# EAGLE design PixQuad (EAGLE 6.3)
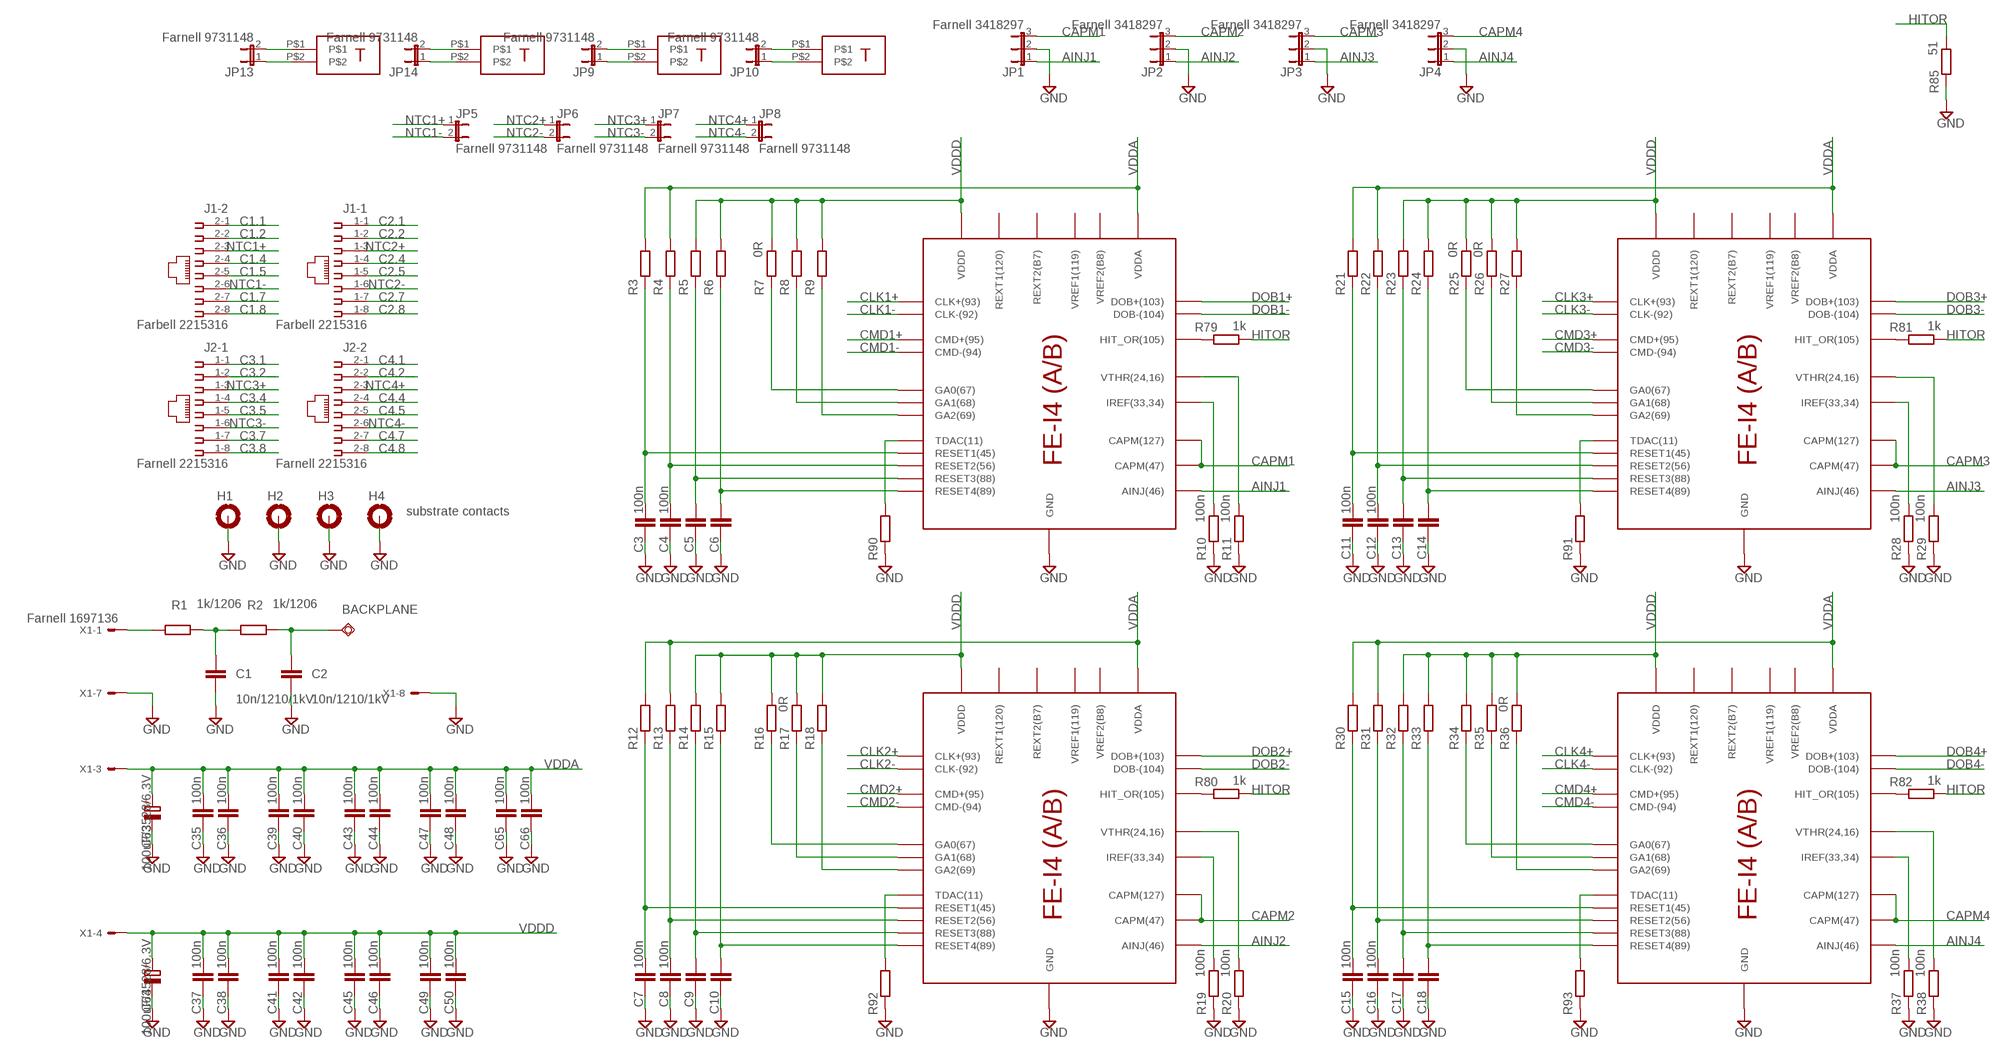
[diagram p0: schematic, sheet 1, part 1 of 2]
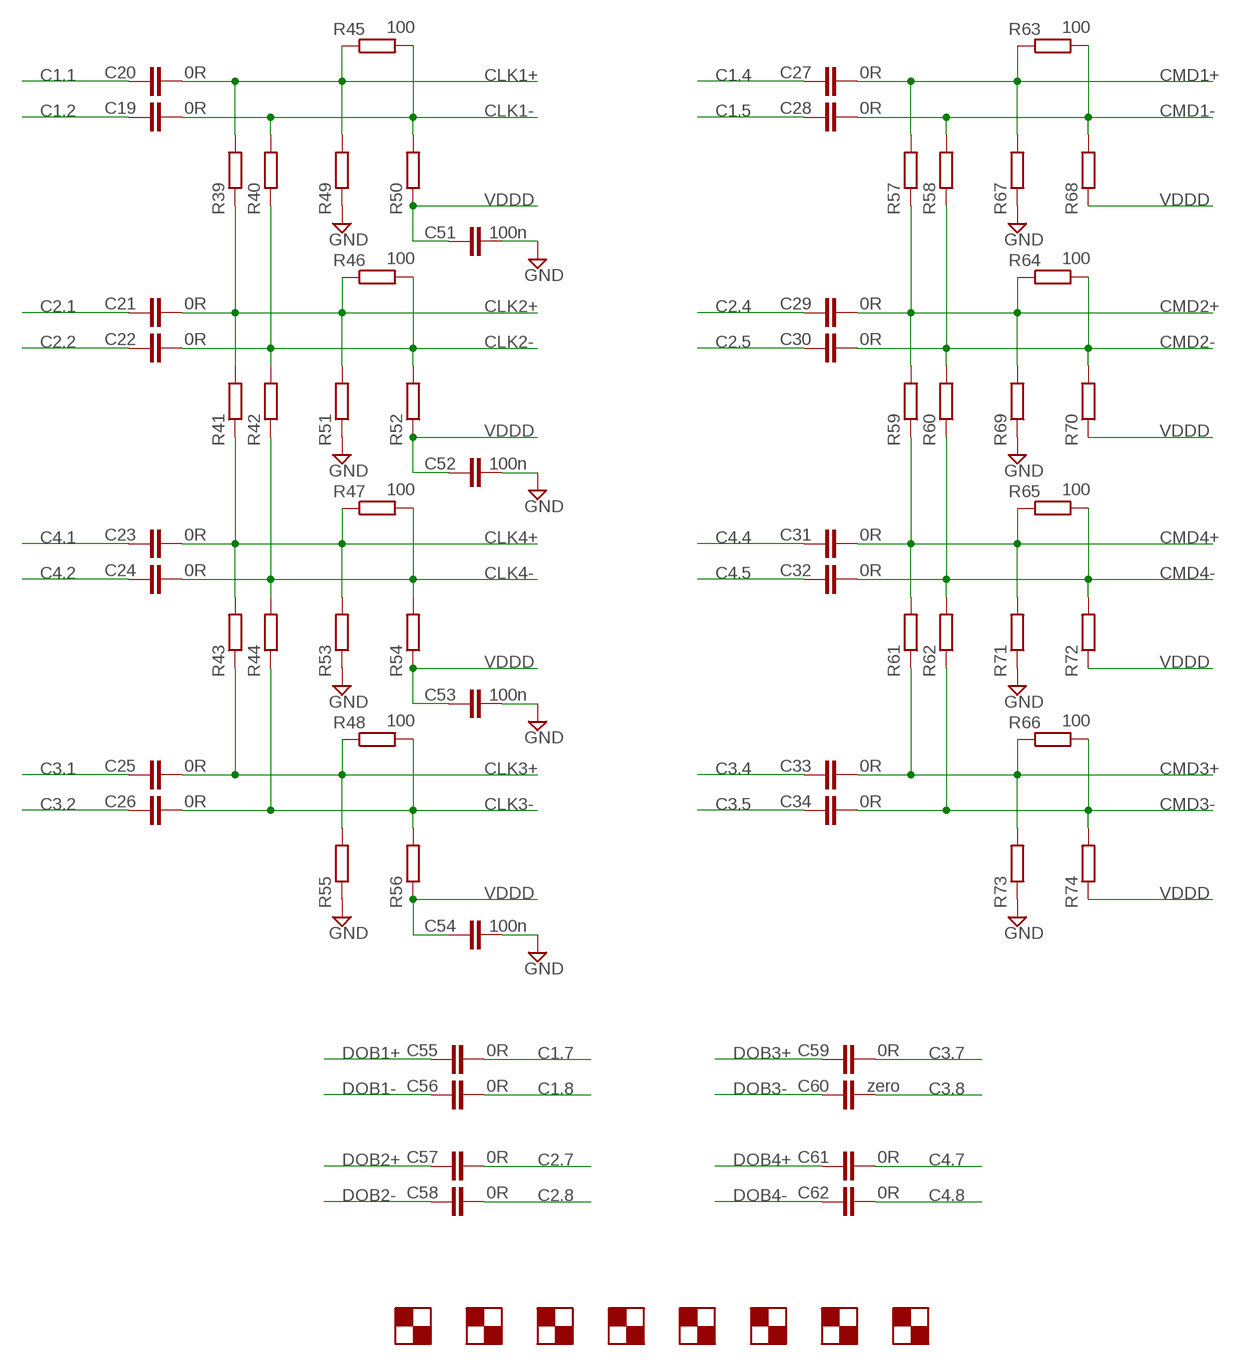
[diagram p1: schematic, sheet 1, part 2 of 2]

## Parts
BACKPLANE  TPSQTP20SQ  [TP20SQ]
C1  10n/1210/1kV  C-EUC1210  [C1210]
C2  10n/1210/1kV  C-EUC1210  [C1210]
C3  100n  C-EUC0402  [C0402]
C4  100n  C-EUC0402  [C0402]
C5  C-EUC0402  [C0402]
C6  C-EUC0402  [C0402]
C7  100n  C-EUC0402  [C0402]
C8  100n  C-EUC0402  [C0402]
C9  C-EUC0402  [C0402]
C10  C-EUC0402  [C0402]
C11  100n  C-EUC0402  [C0402]
C12  100n  C-EUC0402  [C0402]
C13  C-EUC0402  [C0402]
C14  C-EUC0402  [C0402]
C15  100n  C-EUC0402  [C0402]
C16  100n  C-EUC0402  [C0402]
C17  C-EUC0402  [C0402]
C18  C-EUC0402  [C0402]
C19  0R  C-EUC0402  [C0402]
C20  0R  C-EUC0402  [C0402]
C21  0R  C-EUC0402  [C0402]
C22  0R  C-EUC0402  [C0402]
C23  0R  C-EUC0402  [C0402]
C24  0R  C-EUC0402  [C0402]
C25  0R  C-EUC0402  [C0402]
C26  0R  C-EUC0402  [C0402]
C27  0R  C-EUC0402  [C0402]
C28  0R  C-EUC0402  [C0402]
C29  0R  C-EUC0402  [C0402]
C30  0R  C-EUC0402  [C0402]
C31  0R  C-EUC0402  [C0402]
C32  0R  C-EUC0402  [C0402]
C33  0R  C-EUC0402  [C0402]
C34  0R  C-EUC0402  [C0402]
C35  100n  C-EUC0402  [C0402]
C36  100n  C-EUC0402  [C0402]
C37  100n  C-EUC0402  [C0402]
C38  100n  C-EUC0402  [C0402]
C39  100n  C-EUC0402  [C0402]
C40  100n  C-EUC0402  [C0402]
C41  100n  C-EUC0402  [C0402]
C42  100n  C-EUC0402  [C0402]
C43  100n  C-EUC0402  [C0402]
C44  100n  C-EUC0402  [C0402]
C45  100n  C-EUC0402  [C0402]
C46  100n  C-EUC0402  [C0402]
C47  100n  C-EUC0402  [C0402]
C48  100n  C-EUC0402  [C0402]
C49  100n  C-EUC0402  [C0402]
C50  100n  C-EUC0402  [C0402]
C51  100n  C-EUC0402  [C0402]
C52  100n  C-EUC0402  [C0402]
C53  100n  C-EUC0402  [C0402]
C54  100n  C-EUC0402  [C0402]
C55  0R  C-EUC0402  [C0402]
C56  0R  C-EUC0402  [C0402]
C57  0R  C-EUC0402  [C0402]
C58  0R  C-EUC0402  [C0402]
C59  0R  C-EUC0402  [C0402]
C60  zero  C-EUC0402  [C0402]
C61  0R  C-EUC0402  [C0402]
C62  0R  C-EUC0402  [C0402]
C63  100uF/3528/6.3V  CPOL-EUCT3528  [CT3528]
C64  100uF/3528/6.3V  CPOL-EUCT3528  [CT3528]
C65  100n  C-EUC0402  [C0402]
C66  100n  C-EUC0402  [C0402]
H1  MOUNT-PAD-ROUND3.2  [3,2-PAD]
H2  MOUNT-PAD-ROUND3.2  [3,2-PAD]
H3  MOUNT-PAD-ROUND3.2  [3,2-PAD]
H4  substrate contacts  MOUNT-PAD-ROUND3.2  [3,2-PAD]
J1  Farbell 2215316  557560-1  [557560-1]
J2  Farnell 2215316  557560-1  [557560-1]
JP1  Farnell 3418297  JP2E  [JP2]
JP2  Farnell 3418297  JP2E  [JP2]
JP3  Farnell 3418297  JP2E  [JP2]
JP4  Farnell 3418297  JP2E  [JP2]
JP5  Farnell 9731148  JP1E  [JP1]
JP6  Farnell 9731148  JP1E  [JP1]
JP7  Farnell 9731148  JP1E  [JP1]
JP8  Farnell 9731148  JP1E  [JP1]
JP9  Farnell 9731148  JP1E  [JUMPER_JP1]
JP10  Farnell 9731148  JP1E  [JUMPER_JP1]
JP13  Farnell 9731148  JP1E  [JUMPER_JP1]
JP14  Farnell 9731148  JP1E  [JUMPER_JP1]
R1  1k/1206  R-EU_R1206  [R1206]
R2  1k/1206  R-EU_R1206  [R1206]
R3  R-EU_R0402  [R0402]
R4  R-EU_R0402  [R0402]
R5  R-EU_R0402  [R0402]
R6  R-EU_R0402  [R0402]
R7  0R  R-EU_R0402  [R0402]
R8  R-EU_R0402  [R0402]
R9  R-EU_R0402  [R0402]
R10  100n  R-EU_R0402  [R0402]
R11  100n  R-EU_R0402  [R0402]
R12  R-EU_R0402  [R0402]
R13  R-EU_R0402  [R0402]
R14  R-EU_R0402  [R0402]
R15  R-EU_R0402  [R0402]
R16  R-EU_R0402  [R0402]
R17  0R  R-EU_R0402  [R0402]
R18  R-EU_R0402  [R0402]
R19  100n  R-EU_R0402  [R0402]
R20  100n  R-EU_R0402  [R0402]
R21  R-EU_R0402  [R0402]
R22  R-EU_R0402  [R0402]
R23  R-EU_R0402  [R0402]
R24  R-EU_R0402  [R0402]
R25  0R  R-EU_R0402  [R0402]
R26  0R  R-EU_R0402  [R0402]
R27  R-EU_R0402  [R0402]
R28  100n  R-EU_R0402  [R0402]
R29  100n  R-EU_R0402  [R0402]
R30  R-EU_R0402  [R0402]
R31  R-EU_R0402  [R0402]
R32  R-EU_R0402  [R0402]
R33  R-EU_R0402  [R0402]
R34  R-EU_R0402  [R0402]
R35  R-EU_R0402  [R0402]
R36  0R  R-EU_R0402  [R0402]
R37  100n  R-EU_R0402  [R0402]
R38  100n  R-EU_R0402  [R0402]
R39  R-EU_R0402  [R0402]
R40  R-EU_R0402  [R0402]
R41  R-EU_R0402  [R0402]
R42  R-EU_R0402  [R0402]
R43  R-EU_R0402  [R0402]
R44  R-EU_R0402  [R0402]
R45  100  R-EU_R0402  [R0402]
R46  100  R-EU_R0402  [R0402]
R47  100  R-EU_R0402  [R0402]
R48  100  R-EU_R0402  [R0402]
R49  R-EU_R0402  [R0402]
R50  R-EU_R0402  [R0402]
R51  R-EU_R0402  [R0402]
R52  R-EU_R0402  [R0402]
R53  R-EU_R0402  [R0402]
R54  R-EU_R0402  [R0402]
R55  R-EU_R0402  [R0402]
R56  R-EU_R0402  [R0402]
R57  R-EU_R0402  [R0402]
R58  R-EU_R0402  [R0402]
R59  R-EU_R0402  [R0402]
R60  R-EU_R0402  [R0402]
R61  R-EU_R0402  [R0402]
R62  R-EU_R0402  [R0402]
R63  100  R-EU_R0402  [R0402]
R64  100  R-EU_R0402  [R0402]
R65  100  R-EU_R0402  [R0402]
R66  100  R-EU_R0402  [R0402]
R67  R-EU_R0402  [R0402]
R68  R-EU_R0402  [R0402]
R69  R-EU_R0402  [R0402]
R70  R-EU_R0402  [R0402]
R71  R-EU_R0402  [R0402]
R72  R-EU_R0402  [R0402]
R73  R-EU_R0402  [R0402]
R74  R-EU_R0402  [R0402]
R79  1k  R-EU_R0402  [R0402]
R80  1k  R-EU_R0402  [R0402]
R81  1k  R-EU_R0402  [R0402]
R82  1k  R-EU_R0402  [R0402]
R85  51  RCL_R-EU_R0603  [RCL_R0603]
R90  R-EU_R0402  [R0402]
R91  R-EU_R0402  [R0402]
R92  R-EU_R0402  [R0402]
R93  R-EU_R0402  [R0402]
U$1  FE_I4ASIC  [FE-I4]
U$2  FE_I4ASIC  [FE-I4]
U$3  FE_I4ASIC  [FE-I4]
U$4  FE_I4ASIC  [FE-I4]
U$5  AMARK  [AMARK]
U$6  AMARK  [AMARK]
U$7  AMARK  [AMARK]
U$8  AMARK  [AMARK]
U$9  AMARK  [AMARK]
U$10  AMARK  [AMARK]
U$11  AMARK  [AMARK]
U$12  AMARK  [AMARK]
U$17  DORT  [DORT]
U$18  DORT  [DORT]
U$21  DORT  [DORT]
U$22  DORT  [DORT]
X1  Farnell 1697136  FE-I4_5566-8  [FE-I4_5566-8]

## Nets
AINJ1: JP1.1 U$1.AINJ(46)
AINJ2: JP2.1 U$2.AINJ(46)
AINJ3: JP3.1 U$3.AINJ(46)
AINJ4: JP4.1 U$4.AINJ(46)
C1.1: C20.2 J1.2-1
C1.2: C19.2 J1.2-2
C1.4: C27.2 J1.2-4
C1.5: C28.2 J1.2-5
C1.7: C55.1 J1.2-7
C1.8: C56.1 J1.2-8
C2.1: C21.2 J1.1-1
C2.2: C22.2 J1.1-2
C2.4: C29.2 J1.1-4
C2.5: C30.2 J1.1-5
C2.7: C57.1 J1.1-7
C2.8: C58.1 J1.1-8
C3.1: C25.2 J2.1-1
C3.2: C26.2 J2.1-2
C3.4: C33.2 J2.1-4
C3.5: C34.2 J2.1-5
C3.7: C59.1 J2.1-7
C3.8: C60.1 J2.1-8
C4.1: C23.2 J2.2-1
C4.2: C24.2 J2.2-2
C4.4: C31.2 J2.2-4
C4.5: C32.2 J2.2-5
C4.7: C61.1 J2.2-7
C4.8: C62.1 J2.2-8
CAPM1: JP1.3 U$1.CAPM(47) U$1.CAPM(125)(CAPM(127))
CAPM2: JP2.3 U$2.CAPM(47) U$2.CAPM(125)(CAPM(127))
CAPM3: JP3.3 U$3.CAPM(47) U$3.CAPM(125)(CAPM(127))
CAPM4: JP4.3 U$4.CAPM(47) U$4.CAPM(125)(CAPM(127))
CLK1+: C20.1 R39.2 R45.1 R49.2 U$1.CLK+(93)
CLK1-: C19.1 R40.2 R45.2 R50.2 U$1.CLK-(92)
CLK2+: C21.1 R39.1 R41.2 R46.1 R51.2 U$2.CLK+(93)
CLK2-: C22.1 R40.1 R42.2 R46.2 R52.2 U$2.CLK-(92)
CLK3+: C25.1 R43.1 R48.1 R55.2 U$3.CLK+(93)
CLK3-: C26.1 R44.1 R48.2 R56.2 U$3.CLK-(92)
CLK4+: C23.1 R41.1 R43.2 R47.1 R53.2 U$4.CLK+(93)
CLK4-: C24.1 R42.1 R44.2 R47.2 R54.2 U$4.CLK-(92)
CMD1+: C27.1 R57.2 R63.1 R67.2 U$1.CMD+(95)
CMD1-: C28.1 R58.2 R63.2 R68.2 U$1.CMD-(94)
CMD2+: C29.1 R57.1 R59.2 R64.1 R69.2 U$2.CMD+(95)
CMD2-: C30.1 R58.1 R60.2 R64.2 R70.2 U$2.CMD-(94)
CMD3+: C33.1 R61.1 R66.1 R73.2 U$3.CMD+(95)
CMD3-: C34.1 R62.1 R66.2 R74.2 U$3.CMD-(94)
CMD4+: C31.1 R59.1 R61.2 R65.1 R71.2 U$4.CMD+(95)
CMD4-: C32.1 R60.1 R62.2 R65.2 R72.2 U$4.CMD-(94)
DOB1+: C55.2 U$1.DOB+(103)
DOB1-: C56.2 U$1.DOB-(104)
DOB2+: C57.2 U$2.DOB+(103)
DOB2-: C58.2 U$2.DOB-(104)
DOB3+: C59.2 U$3.DOB+(103)
DOB3-: C60.2 U$3.DOB-(104)
DOB4+: C61.2 U$4.DOB+(103)
DOB4-: C62.2 U$4.DOB-(104)
GND: C1.2 C2.2 C3.2 C4.2 C5.2 C6.2 C7.2 C8.2 C9.2 C10.2 C11.2 C12.2 C13.2 C14.2 C15.2 C16.2 C17.2 C18.2 C35.2 C36.2 C37.2 C38.2 C39.2 C40.2 C41.2 C42.2 C43.2 C44.2 C45.2 C46.2 C47.2 C48.2 C49.2 C50.2 C51.1 C52.1 C53.1 C54.1 C63.- C64.- C65.2 C66.2 H1.B3,2(MOUNT) H2.B3,2(MOUNT) H3.B3,2(MOUNT) H4.B3,2(MOUNT) JP1.2 JP2.2 JP3.2 JP4.2 R10.1 R11.1 R19.1 R20.1 R28.1 R29.1 R37.1 R38.1 R49.1 R51.1 R53.1 R55.1 R67.1 R69.1 R71.1 R73.1 R85.1 R90.1 R91.1 R92.1 R93.1 U$1.GND U$2.GND U$3.GND U$4.GND X1.7 X1.8
HITOR: R79.2 R80.2 R81.2 R82.2 R85.2
N$1: BACKPLANE.TP C2.1 R2.2
N$2: C1.1 R1.2 R2.1
N$3: JP13.2 U$17.P$1
N$4: C3.1 R3.1 U$1.RESET1(45)
N$5: C4.1 R4.1 U$1.RESET2(56)
N$6: C5.1 R5.1 U$1.RESET3(88)
N$7: C6.1 R6.1 U$1.RESET4(89)
N$8: R7.1 U$1.GA0(67)
N$9: R8.1 U$1.GA1(68)
N$10: R9.1 U$1.GA2(69)
N$11: R10.2 U$1.IREF(33,34)
N$12: R11.2 U$1.VTHR(24,16)
N$13: R79.1 U$1.HITOR(105)(HIT_OR(105))
N$14: R16.1 U$2.GA0(67)
N$15: R17.1 U$2.GA1(68)
N$16: R18.1 U$2.GA2(69)
N$17: C7.1 R12.1 U$2.RESET1(45)
N$18: C8.1 R13.1 U$2.RESET2(56)
N$19: C9.1 R14.1 U$2.RESET3(88)
N$20: C10.1 R15.1 U$2.RESET4(89)
N$21: R80.1 U$2.HITOR(105)(HIT_OR(105))
N$22: R81.1 U$3.HITOR(105)(HIT_OR(105))
N$23: R82.1 U$4.HITOR(105)(HIT_OR(105))
N$24: R90.2 U$1.TDAC(11)
N$25: R19.2 U$2.IREF(33,34)
N$26: R20.2 U$2.VTHR(24,16)
N$27: R91.2 U$3.TDAC(11)
N$28: R92.2 U$2.TDAC(11)
N$29: R93.2 U$4.TDAC(11)
N$30: JP13.1 U$17.P$2
N$31: JP14.1 U$18.P$2
N$32: JP14.2 U$18.P$1
N$34: R1.1 X1.1
N$46: JP9.1 U$21.P$2
N$47: JP9.2 U$21.P$1
N$48: JP10.1 U$22.P$2
N$49: JP10.2 U$22.P$1
N$50: R27.1 U$3.GA2(69)
N$56: R28.2 U$3.IREF(33,34)
N$57: R26.1 U$3.GA1(68)
N$58: R25.1 U$3.GA0(67)
N$59: C11.1 R21.1 U$3.RESET1(45)
N$60: C12.1 R22.1 U$3.RESET2(56)
N$61: C13.1 R23.1 U$3.RESET3(88)
N$62: C14.1 R24.1 U$3.RESET4(89)
N$64: R29.2 U$3.VTHR(24,16)
N$73: R34.1 U$4.GA0(67)
N$74: R35.1 U$4.GA1(68)
N$75: R36.1 U$4.GA2(69)
N$76: C15.1 R30.1 U$4.RESET1(45)
N$77: C16.1 R31.1 U$4.RESET2(56)
N$78: C17.1 R32.1 U$4.RESET3(88)
N$79: C18.1 R33.1 U$4.RESET4(89)
N$80: R37.2 U$4.IREF(33,34)
N$81: R38.2 U$4.VTHR(24,16)
NTC1+: J1.2-3 JP5.1
NTC1-: J1.2-6 JP5.2
NTC2+: J1.1-3 JP6.1
NTC2-: J1.1-6 JP6.2
NTC3+: J2.1-3 JP7.1
NTC3-: J2.1-6 JP7.2
NTC4+: J2.2-3 JP8.1
NTC4-: J2.2-6 JP8.2
VDDA: C35.1 C36.1 C39.1 C40.1 C43.1 C44.1 C47.1 C48.1 C63.+ C65.1 C66.1 R3.2 R4.2 R12.2 R13.2 R21.2 R22.2 R30.2 R31.2 U$1.VDDA U$2.VDDA U$3.VDDA U$4.VDDA X1.3
VDDD: C37.1 C38.1 C41.1 C42.1 C45.1 C46.1 C49.1 C50.1 C51.2 C52.2 C53.2 C54.2 C64.+ R5.2 R6.2 R7.2 R8.2 R9.2 R14.2 R15.2 R16.2 R17.2 R18.2 R23.2 R24.2 R25.2 R26.2 R27.2 R32.2 R33.2 R34.2 R35.2 R36.2 R50.1 R52.1 R54.1 R56.1 R68.1 R70.1 R72.1 R74.1 U$1.VDDD U$2.VDDD U$3.VDDD U$4.VDDD X1.4
Unconnected: U$1.REXT1(120) U$1.REXT2(B7) U$1.VREF1(119) U$1.VREF2(B8) U$2.REXT1(120) U$2.REXT2(B7) U$2.VREF1(119) U$2.VREF2(B8) U$3.REXT1(120) U$3.REXT2(B7) U$3.VREF1(119) U$3.VREF2(B8) U$4.REXT1(120) U$4.REXT2(B7) U$4.VREF1(119) U$4.VREF2(B8)

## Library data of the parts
BACKPLANE = testpad:TPSQ: Test pad
C1-C62 C65 C66 = rcl:C-EU: CAPACITOR, European symbol
C63 C64 = rcl:CPOL-EU: POLARIZED CAPACITOR, European symbol
H1-H4 = holes:MOUNT-PAD-ROUND: MOUNTING PAD, round
J1 J2 = con-amp:557560-1: AMP connector
JP1-JP4 = jumper:JP2E: JUMPER
JP5-JP8 = jumper:JP1E: JUMPER
JP9 JP10 JP13 JP14 = FE-I4:JP1E: JUMPER
R1-R74 R79-R82 R90-R93 = rcl:R-EU_: RESISTOR, European symbol
R85 = FE-I4:RCL_R-EU_: RESISTOR, European symbol
U$1-U$4 = FE-I4:FE_I4
U$5-U$12 = FE-I4:AMARK
U$17 U$18 U$21 U$22 = FE-I4:DORT
X1 = FE-I4:FE-I4_5566-8: Mini FIT connector 8 pol Source: http://www.molex.com; OC_FARNELL: unknown; OC_NEWARK: unknown

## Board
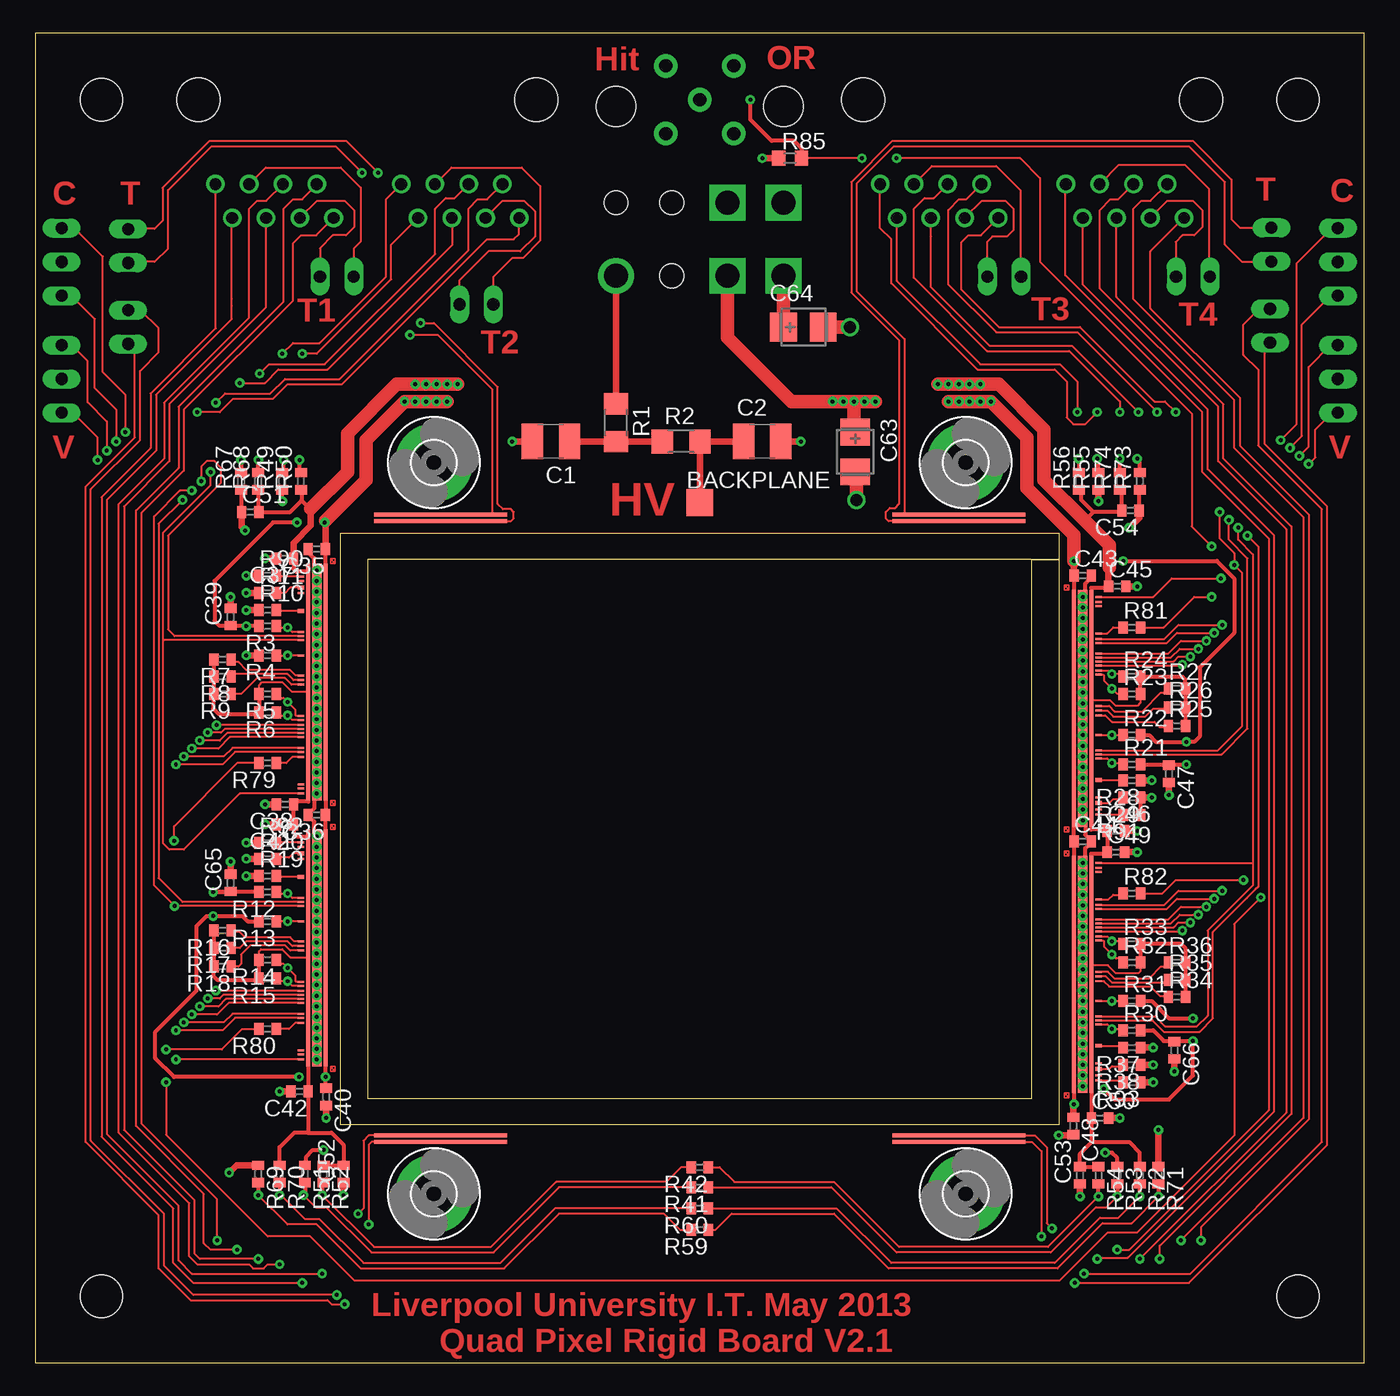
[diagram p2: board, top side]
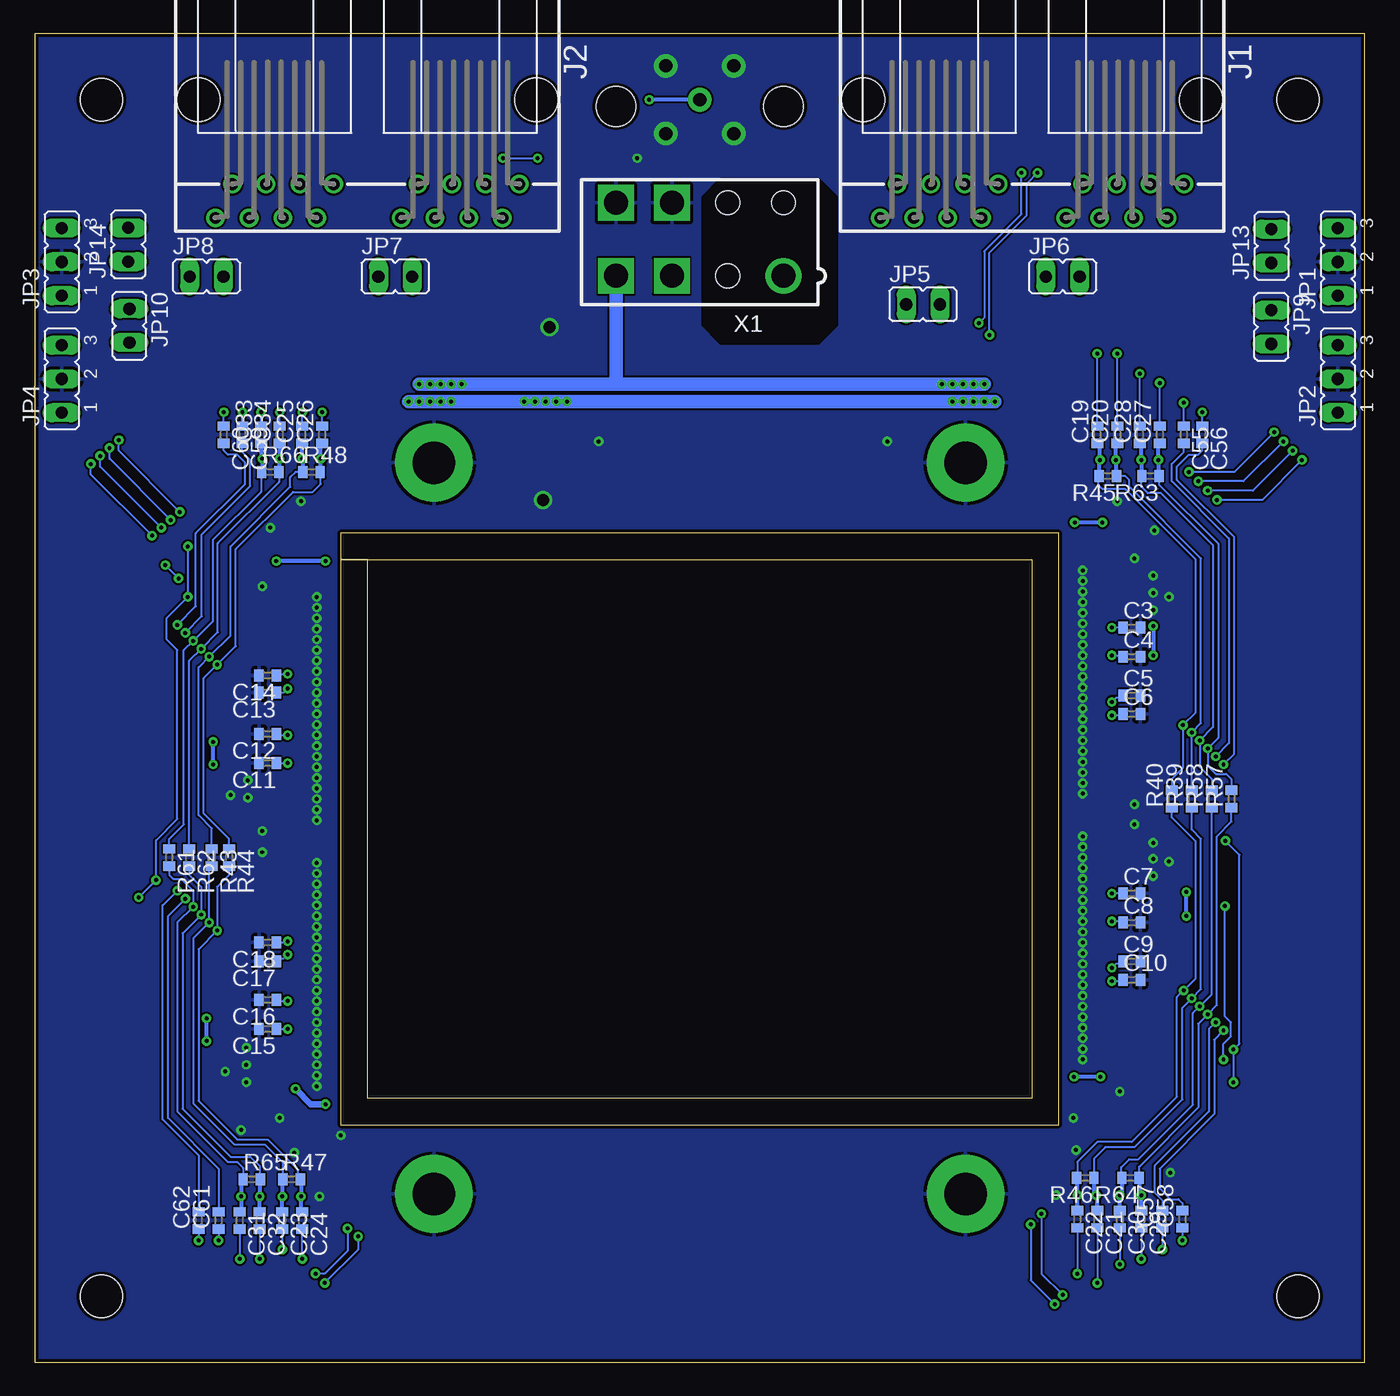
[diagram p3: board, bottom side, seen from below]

Size 100 x 100 mm. Coordinates in mm from the lower left corner, seen from the top.
Outline: 0,0 100,0 100,100 0,100 0,0
Copper layers (1+2*15+16): Top 0.035mm / dielectric 1.5mm / Route2 0.035mm / dielectric 0.15mm / Route15 0.035mm / dielectric 0.2mm / Bottom 0.035mm
Design rules "default *": minimum track width 10mil, minimum drill 24mil, track to track 6mil, track to pad 6mil, pad to pad 6mil, via to via 6mil, smd to smd 6mil, copper to edge 10mil, drill to drill 8mil, minimum pad ring 10mil, minimum via ring 8mil, stop-mask expansion 4mil, vias tented up to drill 0mil, thermal gap 10mil
Holes 3.2 mm at 5,5 5,95 95,95 95,5

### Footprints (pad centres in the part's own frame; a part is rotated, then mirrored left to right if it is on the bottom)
TP20SQ = smd 2 x 2: TP 0,0
C1210 = smd 1.6 x 2.7: 1 -1.4,0; 2 1.4,0
C0402 = smd 0.7 x 0.9: 1 -0.65,0; 2 0.65,0
CT3528 = smd 2 x 2.2: + -1.5,0; - 1.5,0
3,2-PAD = drill 3.2 pad 5.842: B3,2 0,0
557560-1 = drill 0.889: 1-1 -11.43,6.35; 1-2 -10.16,8.89; 1-3 -8.89,6.35; 1-4 -7.62,8.89; 1-5 -6.35,6.35; 1-6 -5.08,8.89; 1-7 -3.81,6.35; 1-8 -2.54,8.89; 2-1 2.54,6.35; 2-2 3.81,8.89; 2-3 5.08,6.35; 2-4 6.35,8.89; 2-5 7.62,6.35; 2-6 8.89,8.89; 2-7 10.16,6.35; 2-8 11.43,8.89 | hole 3.251: -12.7,0; 12.7,0
JP2 = drill 0.914 long: 1 -2.54,0; 2 0,0; 3 2.54,0
JP1 = drill 0.914 long: 1 0,-1.27; 2 0,1.27
JUMPER_JP1 = drill 0.914 long: 1 0,-1.27; 2 0,1.27
R1206 = smd 1.6 x 1.803: 1 -1.422,0; 2 1.422,0
R0402 = smd 0.7 x 0.9: 1 -0.65,0; 2 0.65,0
RCL_R0603 = smd 1 x 1.1: 1 -0.85,0; 2 0.85,0
FE-I4 = smd 0.15 x 0.5: AINJ(46) -4.45,-2; CAPM(47) -4.15,-2; CAPM(125) 7.4,-2; CLK+(93) 2.55,-2; CLK-(92) 2.25,-2; CMD+(95) 3.15,-2; CMD-(94) 2.85,-2; DOB+(103) 3.95,-2; DOB-(104) 4.25,-2; GA0(67) -1.5,-2; GA1(68) -1.15,-2; GA2(69) -0.8,-2; HITOR(105) 4.65,-2; RESET1(45) -4.75,-2; RESET2(56) -3,-2; RESET3(88) 1.55,-2; RESET4(89) 1.85,-2; REXT1(120) 7,-2; REXT2(B7) -8.6,-2; TDAC(11) -8.95,-2; VREF1(119) 6.7,-2; VREF2(B8) -7.7,-2 | smd 17.8 x 0.7: GND -1,-0.8 | smd 0.3 x 0.5: IREF(33,34) -6.35,-2; VTHR(24,16) -8.1,-2 | smd 17.8 x 0.3: VDDA -1,-0.15; VDDD -1,-1.45
DORT = smd 10 x 0.3: P$1 5,0; P$2 5,0.5
FE-I4_5566-8 = drill 1.8: 1 6.3,-2.75 | drill 1.8 square: 3 -2.1,-2.75; 4 -6.3,-2.75; 7 -2.1,2.75; 8 -6.3,2.75 | hole 1.8: 2.1,-2.75; 2.1,2.75; 6.3,2.75 | hole 3: -6.3,10; 6.3,10

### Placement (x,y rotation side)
BACKPLANE  50,64.7 0 top
C1  38.8,69.3 180 top
C2  54.7,69.3 0 top
C3  17.5,55.3 0 bottom
C4  17.5,53.1 0 bottom
C5  17.5,50.2 0 bottom
C6  17.5,48.8 0 bottom
C7  17.5,35.3 0 bottom
C8  17.5,33.1 0 bottom
C9  17.5,30.2 0 bottom
C10  17.5,28.8 0 bottom
C11  82.5,45.1 180 bottom
C12  82.5,47.3 180 bottom
C13  82.5,50.4 180 bottom
C14  82.5,51.7 180 bottom
C15  82.5,25.1 180 bottom
C16  82.5,27.3 180 bottom
C17  82.5,30.2 180 bottom
C18  82.5,31.6 180 bottom
C19  20.1,69.8 90 bottom
C20  18.6,69.8 90 bottom
C21  20.1,10.8 270 bottom
C22  21.6,10.8 270 bottom
C23  81.4,10.7 270 bottom
C24  79.9,10.7 270 bottom
C25  79.9,69.8 90 bottom
C26  78.4,69.8 90 bottom
C27  15.4,69.8 90 bottom
C28  16.9,69.8 90 bottom
C29  16.8,10.8 270 bottom
C30  18.4,10.8 270 bottom
C31  84.6,10.7 270 bottom
C32  83.1,10.7 270 bottom
C33  83,69.8 90 bottom
C34  81.6,69.8 90 bottom
C35  21.2,61.2 180 top
C36  21.2,41.2 180 top
C37  18.8,60.5 180 top
C38  18.8,42 180 top
C39  14.7,56.1 90 top
C40  21.9,20 270 top
C41  18.8,40.5 180 top
C42  19.9,20.4 180 top
C43  78.8,59.2 0 top
C44  78.8,39.2 0 top
C45  81.4,58.4 0 top
C46  81.3,40 0 top
C47  85.3,44.3 270 top
C48  78.1,17.8 270 top
C49  81.3,38.4 0 top
C50  80.1,18.4 0 top
C51  16.2,64 0 top
C52  23.2,14.2 90 top
C53  78.6,14.1 90 top
C54  82.4,64.1 180 top
C55  13.6,69.8 270 bottom
C56  12.2,69.8 270 bottom
C57  15.2,10.8 90 bottom
C58  13.7,10.8 90 bottom
C59  84.4,69.8 270 bottom
C60  85.8,69.8 270 bottom
C61  86.2,10.7 90 bottom
C62  87.7,10.7 90 bottom
C63  61.7,68.5 270 top
C64  57.8,77.9 0 top
C65  14.7,36.1 90 top
C66  85.7,23.5 270 top
H1  30,67.7 0 top
H2  30,12.7 0 top
H3  70,67.7 0 top
H4  70,12.7 0 top
J1  25,95 180 bottom
J2  75,95 180 bottom
JP1  2,82.8 90 bottom
JP2  2,74 90 bottom
JP3  98,82.8 90 bottom
JP4  98,74 90 bottom
JP5  33.2,79.6 270 bottom
JP6  22.7,81.7 270 bottom
JP7  72.9,81.7 270 bottom
JP8  87.1,81.7 270 bottom
JP9  7,77.9 180 bottom
JP10  92.9,78 180 bottom
JP13  7,84 0 bottom
JP14  93,84.1 0 bottom
R1  43.7,70.7 270 top
R2  48.6,69.3 0 top
R3  17.5,55.4 180 top
R4  17.5,53.2 180 top
R5  17.5,50.3 180 top
R6  17.5,48.9 180 top
R7  14.1,52.9 180 top
R8  14.1,51.6 180 top
R9  14.1,50.3 180 top
R10  17.5,56.6 0 top
R11  17.5,57.9 0 top
R12  17.5,35.4 180 top
R13  17.5,33.2 180 top
R14  17.5,30.3 180 top
R15  17.5,28.9 180 top
R16  14.1,32.5 180 top
R17  14.1,31.2 180 top
R18  14.1,29.8 180 top
R19  17.5,36.6 0 top
R20  17.5,37.9 0 top
R21  82.5,45 0 top
R22  82.5,47.2 0 top
R23  82.5,50.3 0 top
R24  82.5,51.6 0 top
R25  85.9,47.9 0 top
R26  85.9,49.3 0 top
R27  85.9,50.7 0 top
R28  82.5,43.8 180 top
R29  82.5,42.5 180 top
R30  82.5,25 0 top
R31  82.5,27.2 0 top
R32  82.5,30.1 0 top
R33  82.5,31.5 0 top
R34  85.9,27.5 0 top
R35  85.9,28.8 0 top
R36  85.9,30.1 0 top
R37  82.5,23.7 180 top
R38  82.5,22.4 180 top
R39  13,42.4 90 bottom
R40  14.5,42.4 90 bottom
R41  50,13.2 180 top
R42  50,14.7 180 top
R43  86.7,38 270 bottom
R44  85.4,38 270 bottom
R45  19.3,66.7 180 bottom
R46  21,13.9 180 bottom
R47  80.7,13.8 0 bottom
R48  79.2,67 0 bottom
R49  18.6,66.3 90 top
R50  20,66.3 90 top
R51  20.3,14.2 270 top
R52  21.7,14.2 270 top
R53  81.4,14.1 270 top
R54  80,14.1 270 top
R55  80,66.3 90 top
R56  78.5,66.3 90 top
R57  10,42.4 90 bottom
R58  11.5,42.4 90 bottom
R59  50,10 180 top
R60  50,11.6 180 top
R61  89.9,38 270 bottom
R62  88.4,38 270 bottom
R63  16.1,66.7 180 bottom
R64  17.6,13.9 180 bottom
R65  83.7,13.8 0 bottom
R66  82.3,67 0 bottom
R67  15.5,66.3 90 top
R68  16.8,66.3 90 top
R69  16.8,14.2 270 top
R70  18.4,14.2 270 top
R71  84.5,14.1 270 top
R72  83.1,14.1 270 top
R73  83.1,66.3 90 top
R74  81.6,66.3 90 top
R79  17.5,45.1 180 top
R80  17.5,25.1 180 top
R81  82.5,55.3 0 top
R82  82.5,35.3 0 top
R85  56.8,90.6 0 top
R90  17.5,59.2 0 top
R91  82.5,41.2 180 top
R92  17.5,39.1 0 top
R93  82.5,21.1 180 top
U$1  22,50.2 270 top
U$2  22,30.2 270 top
U$3  78,50.2 90 top
U$4  78,30.2 90 top
U$5  22.4,22.1 0 top
U$6  22.4,40.3 0 top
U$7  22.4,42.1 0 top
U$8  22.4,60.3 0 top
U$9  77.6,58.3 0 top
U$10  77.6,40.1 0 top
U$11  77.6,38.3 0 top
U$12  77.6,20.1 0 top
U$17  25.5,63.3 0 top
U$18  64.5,63.3 0 top
U$21  25.5,16.6 0 top
U$22  64.5,16.6 0 top
X1  50,84.5 0 bottom

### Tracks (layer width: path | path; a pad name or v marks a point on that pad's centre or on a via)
AINJ1  (via drill 0.3)
  Top 0.15: U$1.AINJ(46) 10.5,54.65 10,55.15 10,62.2 14,66.2 14,67.3 13.5,67.8 12.9,67.8 12.5,67.4 v12.5,66.3 | v6.1,69.3 6.1,71.7 4.5,73.3 4.5,78.5 2.74,80.26 JP1.1
  Bottom 0.15: v6.1,69.3 9.1,66.3 v12.5,66.3
AINJ2  (via drill 0.3)
  Top 0.15: U$2.AINJ(46) 11.1,34.65 9.3,36.45 9.3,63.1 v11.1,64.9 | v4.7,67.9 4.7,69.6 2.84,71.46 JP2.1
  Bottom 0.15: v4.7,67.9 7.7,64.9 v11.1,64.9
AINJ3  (via drill 0.3)
  Top 0.15: U$3.AINJ(46) 89.25,45.75 91.2,47.7 91.2,60.5 89.8,61.9 v89.8,63.4 | v94.4,68.8 95.3,69.7 95.3,78.1 97.46,80.26 JP3.1
  Bottom 0.15: v89.8,63.4 94.4,68 v94.4,68.8
AINJ4  (via drill 0.3)
  Top 0.15: U$4.AINJ(46) 84.05,25.75 84.9,24.9 87.6,24.9 88.6,25.9 88.6,32.4 91.15,34.95 91.8,35.6 92,35.8 92,61.4 v91.2,62.2 | v95.8,67.6 96.3,68.1 96.3,70.2 97.56,71.46 JP4.1
  Bottom 0.15: v91.2,62.2 95.8,66.8 v95.8,67.6
C1.1  (via drill 0.3)
  Top 0.15: v18.6,75.9 19.4,76.7 21.4,76.7 26.4,81.7 26.4,87.51 J1.2-1 27.5,88.61
  Bottom 0.15: C20.2 v18.6,75.9
C1.2  (via drill 0.3)
  Top 0.15: J1.2-2 26.8,84.1 26.8,81.5 21.2,75.9 v20.1,75.9
  Bottom 0.15: C19.2 v20.1,75.9
C1.4  (via drill 0.3)
  Top 0.15: v15.4,73.7 17.3,73.7 18.3,74.7 22,74.7 31.4,84.1 31.4,86.06 J1.2-4
  Bottom 0.15: C27.2 v15.4,73.7
C1.5  (via drill 0.3)
  Top 0.15: v16.9,74.4 17.6,75.1 21.8,75.1 30.1,83.4 30.1,86.8 30.9,87.6 31.57,87.6 J1.2-5
  Bottom 0.15: C28.2 v16.9,74.4
C1.7  (via drill 0.3)
  Top 0.15: v13.6,72.2 14.3,72.9 17.7,72.9 18.8,74 22.9,74 32.6,83.7 32.6,86.8 33.3,87.5 34.01,87.5 J1.2-7
  Bottom 0.15: C55.1 v13.6,72.2
C1.8  (via drill 0.3)
  Top 0.15: v12.2,71.5 13.9,71.5 14.9,72.5 17.9,72.5 19,73.6 23.1,73.6 34,84.5 36,84.5 36.4,84.9 36.4,86.08 J1.2-8
  Bottom 0.15: C56.1 v12.2,71.5
C2.1  (via drill 0.3)
  Top 0.15: J1.1-1 13.6,88.62 13.6,77.8 8.7,72.9 8.7,68.8 5,65.1 5,17 10.4,11.6 10.4,7.5 11.9,6 v20.1,6
  Bottom 0.15: C21.2 v20.1,6
C2.2  (via drill 0.3)
  Top 0.15: J1.1-2 14.8,86.07 14.8,80 14.8,79.5 14.8,78.5 9.1,72.8 9.1,68.6 5.4,64.9 5.4,17.2 10.8,11.8 10.8,7.7 11.8,6.7 v21.6,6.7
  Bottom 0.15: C22.2 v21.6,6.7
C2.4  (via drill 0.3)
  Top 0.15: v16.8,7.8 12.4,7.8 12,8.2 12,12.2 6.7,17.5 6.7,64.4 10.1,67.8 10.1,72.1 17.38,79.38 17.38,80.38 17.38,80.9 J1.1-4
  Bottom 0.15: C29.2 v16.8,7.8
C2.5  (via drill 0.3)
  Top 0.15: v18.4,7.4 17.5,7.4 17.2,7.1 16.4,7.1 16.1,7.4 12.2,7.4 11.6,8 11.6,12 6.3,17.3 6.3,64.6 9.7,68 9.7,72.2 16.1,78.6 16.1,86.8 16.7,87.4 17.4,87.4 J1.1-5
  Bottom 0.15: C30.2 v18.4,7.4
C2.7  (via drill 0.3)
  Top 0.15: v15.2,8.5 13.2,8.5 12.7,9 12.7,12.7 7.6,17.8 7.6,64.1 10.8,67.3 10.8,71.9 18.7,79.8 18.7,86.8 19.4,87.5 20.1,87.5 21.19,88.59 J1.1-7
  Bottom 0.15: C57.1 v15.2,8.5
C2.8  (via drill 0.3)
  Top 0.15: J1.1-8 21.15,84.8 20,84.8 19.4,84.2 19.4,81 19.4,80.7 19.4,79.9 11.2,71.7 11.2,67.1 8,63.9 8,18 13.7,12.3 v13.7,9.2
  Bottom 0.15: C58.1 v13.7,9.2
C3.1  (via drill 0.3)
  Top 0.15: v79.9,71.5 79,70.6 78.1,70.6 77.6,71.1 77.6,73.8 76.7,74.7 70.9,74.7 64.4,81.2 64.4,84.5 63.57,85.33 J2.1-1
  Bottom 0.15: C25.2 v79.9,71.5
C3.2  (via drill 0.3)
  Top 0.15: J2.1-2 64.84,81.36 71.1,75.1 77.1,75.1 78.4,73.8 v78.4,71.5
  Bottom 0.15: C26.2 v78.4,71.5
C3.4  (via drill 0.3)
  Top 0.15: J2.1-4 67.38,84.72 67.4,84.7 67.4,80.9 71.8,76.5 78,76.5 v83,71.5
  Bottom 0.15: C33.2 v83,71.5
C3.5  (via drill 0.3)
  Top 0.15: v81.6,71.5 81.6,72.3 77.8,76.1 71.6,76.1 66.1,81.6 66.1,86.8 66.9,87.6 67.6,87.6 J2.1-5
  Bottom 0.15: C34.2 v81.6,71.5
C3.7  (via drill 0.3)
  Top 0.15: v84.4,71.5 78.4,77.5 72.3,77.5 68.7,81.1 68.7,86.7 69.5,87.5 70.04,87.5 J2.1-7
  Bottom 0.15: C59.1 v84.4,71.5
C3.8  (via drill 0.3)
  Top 0.15: v85.8,71.5 85,72.3 84.2,72.3 78.6,77.9 72.5,77.9 69.7,80.7 69.7,84.3 70.2,84.8 71.15,84.8 J2.1-8 72.5,86.07
  Bottom 0.15: C60.1 v85.8,71.5
C4.1  (via drill 0.3)
  Top 0.15: v81.4,8.5 82.3,8.5 92.8,19 92.8,62 87.8,67 87.8,71.5 77.5,81.8 77.5,82.8 77.5,83 77.5,88.61 J2.2-1
  Bottom 0.15: C23.2 v81.4,8.5
C4.2  (via drill 0.3)
  Top 0.15: v79.9,7.8 80,7.9 82.2,7.9 93.2,18.9 93.2,62.2 88.2,67.2 88.2,71.7 78.81,81.09 J2.2-2
  Bottom 0.15: v79.9,7.8 C24.2
C4.4  (via drill 0.3)
  Top 0.15: v84.6,7.8 84.6,8.8 94.5,18.7 94.5,62.9 89.4,68 89.4,72.1 81.35,80.15 J2.2-4
  Bottom 0.15: C31.2 v84.6,7.8
C4.5  (via drill 0.3)
  Top 0.15: v83.1,7.8 94.1,18.8 94.1,62.7 89,67.8 89,71.9 80.1,80.8 80.1,86.7 80.9,87.5 81.47,87.5 J2.2-5
  Bottom 0.15: C32.2 v83.1,7.8
C4.7  (via drill 0.3)
  Top 0.15: v86.2,9.2 95.4,18.4 95.4,63.6 90.2,68.8 90.2,72.4 82.6,80 82.6,86.8 83.2,87.4 83.91,87.4 J2.2-7
  Bottom 0.15: C61.1 v86.2,9.2
C4.8  (via drill 0.3)
  Top 0.15: J2.2-8 86.41,86.11 83.9,83.6 83.9,79.3 90.65,72.55 90.65,68.95 95.8,63.8 95.8,18.3 87.7,10.2 v87.7,9.2
  Bottom 0.15: C62.1 v87.7,9.2
CAPM1  (via drill 0.3)
  Top 0.15: U$1.CAPM(47) 9.7,54.35 9.65,54.4 | v13.2,67 13.2,66 9.65,62.45 9.65,54.4 | v6.8,70 6.8,72.8 5.1,74.5 5.1,83.2 2.96,85.34 JP1.3 | U$1.CAPM(125) 15.4,42.8 11.2,38.6 10.1,38.6 9.65,39.05 9.65,54.4
  Bottom 0.15: v6.8,70 9.8,67 v13.2,67
CAPM2  (via drill 0.3)
  Top 0.15: v11.8,65.6 10.9,65.6 8.95,63.65 8.95,35.9 v10.5,34.35 U$2.CAPM(47) | v5.4,68.6 5.4,70.8 3.95,72.25 3.95,75.35 2.76,76.54 JP2.3 | U$2.CAPM(125) v10.6,22.8
  Bottom 0.15: v5.4,68.6 8.4,65.6 v11.8,65.6 | v10.6,22.8 10.6,24 10.05,24.55 10.05,25.6 10.5,26.05 v10.5,34.35
CAPM3  (via drill 0.3)
  Top 0.15: U$3.CAPM(47) 88.95,46.05 90.8,47.9 90.8,59.4 v90.2,60 90.2,60.9 89.1,62 v89.1,64 | v93.7,69.4 94.9,70.6 94.9,82.7 97.54,85.34 JP3.3 | U$3.CAPM(125) 84.1,57.6 85.5,59 v89.2,59
  Bottom 0.15: v89.1,64 93.7,68.6 v93.7,69.4 | v89.2,59 v90.2,60
CAPM4  (via drill 0.3)
  Top 0.15: U$4.CAPM(47) 84.25,26.05 85,25.3 87.4,25.3 88.2,26.1 88.2,32.5 91.6,35.9 91.6,37.6 | v90.5,62.8 90.5,61.9 91.6,60.8 91.6,37.6 | v95.1,68.2 95.8,68.9 95.8,74.9 97.44,76.54 JP4.3 | U$4.CAPM(125) 91.6,37.6
  Bottom 0.15: v90.5,62.8 95.1,67.4 v95.1,68.2
CLK1+  (via drill 0.3)
  Top 0.15: U$1.CLK+(93) 14.25,47.65 14,47.4 v13,47.4
  Top 0.3: R49.2 18.7,66.95 v18.7,67.9
  Bottom 0.15: R39.2 v13,47.4 12.3,48.1 12.3,60.5 17.7,65.9 17.7,66.4 18,66.7 R45.1 18.65,66.9 R49.2
  Bottom 0.3: C20.1 18.7,69.05 v18.7,67.9 18.65,67.85 R45.1
CLK1-  (via drill 0.3)
  Top 0.15: U$1.CLK-(92) v13.65,47.95
  Top 0.3: R50.2 19.9,66.95 v19.9,67.9
  Bottom 0.15: R40.2 14.5,43.9 13.65,44.75 v13.65,47.95 12.7,48.9 12.7,60.4 18,65.7 19.7,65.7 20,66 20,66.65 R45.2
  Bottom 0.3: C19.1 19.9,68.95 v19.9,67.9 19.95,67.85 R45.2
CLK2+  (via drill 0.3)
  Top 0.15: U$2.CLK+(93) 14.15,27.65 13.9,27.4 v13,27.4 | R41.2 39.4,13.2 34.5,8.3 25.3,8.3 21.9,11.7 21.1,11.7 v20.2,12.6
  Top 0.3: 20.2,13.45 R51.2 20.3,12.7 v20.2,12.6
  Bottom 0.15: R39.1 13,40.1 12.3,39.4 12.3,28.1 v13,27.4 13.7,26.7 13.7,19.8 17.3,16.2 19.5,16.2 20.35,15.35 R46.1
  Bottom 0.3: R46.1 20.35,12.75 v20.2,12.6 20.1,12.5 C21.1
CLK2-  (via drill 0.3)
  Top 0.15: U$2.CLK-(92) 13.65,27.95 v13.6,28 | R42.2 48.6,14.7 47.5,13.6 39.2,13.6 34.3,8.7 25.5,8.7 v21.6,12.6
  Top 0.3: R52.2 21.6,13.45 v21.6,12.6
  Bottom 0.15: v13.6,28 12.7,28.9 12.7,39.2 14.5,41 R40.1 | v13.6,28 13.7,27.9 | v13.6,28 14.1,27.5 14.1,20 17.5,16.6 20.1,16.6 21.6,15.1 21.6,13.95 R46.2 | 21.65,12.65 v21.6,12.6
  Bottom 0.3: R46.2 21.65,12.65 | C22.1 v21.6,12.6
CLK3+  (via drill 0.3)
  Top 0.15: U$3.CLK+(93) 85.65,52.75 86,53.1 v86.9,53.1
  Top 0.3: R55.2 80,67.9 v79.9,68
  Bottom 0.15: R43.1 86.7,40.2 87.7,41.2 87.7,52.3 v86.9,53.1 85.3,54.7 85.3,61.4 80.8,65.9 80.8,66.6 80.4,67 R48.1
  Bottom 0.3: C25.1 v79.9,68 79.85,67.95 R48.1
CLK3-  (via drill 0.3)
  Top 0.15: U$3.CLK-(92) 86.25,52.45 v86.3,52.5
  Top 0.3: v78.5,68 R56.2
  Bottom 0.15: R44.1 85.4,39.4 87.3,41.3 87.3,51.5 v86.3,52.5 84.9,53.9 84.9,61.2 80.6,65.5 79.1,65.5 78.5,66.1 R56.2 R48.2
  Bottom 0.3: C26.1 78.5,69.05 v78.5,68 78.5,67.05 R48.2
CLK4+  (via drill 0.3)
  Top 0.15: U$4.CLK+(93) 85.65,32.75 86,33.1 v86.9,33.1 | R41.1 59.9,13.2 64.8,8.3 76.4,8.3 79.8,11.7 80.6,11.7 v81.4,12.5
  Top 0.3: R53.2 v81.4,12.5
  Bottom 0.15: R43.2 86.9,37.15 v86.9,33.1 88.1,31.9 88.1,19.5 85,16.4 82.7,16.4 81.35,15.05 R47.1
  Bottom 0.3: C23.1 v81.4,12.5 81.4,13.75 R47.1
CLK4-  (via drill 0.3)
  Top 0.15: U$4.CLK-(92) 86.25,32.45 v86.3,32.5 | R42.1 51.5,14.7 52.6,13.6 60.1,13.6 65,8.7 76.2,8.7 v80,12.5
  Top 0.3: v80,12.5 R54.2
  Bottom 0.15: R44.2 85.4,36.7 86.3,35.8 v86.3,32.5 87.7,31.1 87.7,19.7 84.8,16.8 82.5,16.8 80.2,14.5 80.2,13.95 R47.2
  Bottom 0.3: C24.1 80,11.45 v80,12.5 80,13.75 R47.2
CMD1+  (via drill 0.3)
  Top 0.15: U$1.CMD+(95) 14.65,47.05 13.8,46.2 v11.8,46.2
  Top 0.3: v15.5,67.9 R67.2
  Bottom 0.15: R57.2 10,43.9 10.4,44.3 11.2,44.3 11.8,44.9 v11.8,46.2 11,47 11,61.6 15.45,66.05 R63.1
  Bottom 0.3: C27.1 15.5,69.05 v15.5,67.9 15.45,67.85 R63.1
CMD1-  (via drill 0.3)
  Top 0.15: U$1.CMD-(94) 14.45,47.35 13.9,46.8 v12.4,46.8
  Top 0.3: R68.2 v16.8,67.9
  Bottom 0.15: R58.2 11.5,43.9 12.4,44.8 v12.4,46.8 11.4,47.8 11.4,61.5 15.3,65.4 16.3,65.4 16.8,65.9 16.8,66.65 R63.2
  Bottom 0.3: C28.1 16.8,69.05 v16.8,67.9 16.75,67.85 R63.2
CMD2+  (via drill 0.3, 0.3 pad 0.7)
  Top 0.15: U$2.CMD+(95) 14.55,27.05 13.7,26.2 v11.8,26.2 | R59.2 48.5,10 47.3,11.2 39.4,11.2 35.3,7.1 24.5,7.1 21.2,10.4 19,10.4 v16.8,12.6
  Top 0.3: 17.1,13.45 R69.2 v16.8,12.6
  Bottom 0.15: R57.1 10,40.7 11.1,39.6 11.1,26.9 v11.8,26.2 12.5,25.5 12.5,19.2 16.95,14.75 R64.1
  Bottom 0.3: C29.1 v16.8,12.6 16.95,12.75 R64.1
CMD2-  (via drill 0.3)
  Top 0.15: U$2.CMD-(94) 14.35,27.35 13.8,26.8 v12.4,26.8 | R60.2 39.1,11.6 35,7.5 24.7,7.5 21.4,10.8 20.3,10.8 18.5,12.6 v18.4,12.6
  Top 0.3: 18.6,13.35 R70.2 v18.4,12.6
  Bottom 0.15: v12.4,26.8 11.5,27.7 R58.1 | v12.4,26.8 12.5,26.7 | v12.4,26.8 12.9,26.3 12.9,19.4 17,15.3 17.7,15.3 18.3,14.7 18.3,13.95 R64.2
  Bottom 0.3: R64.2 18.25,12.75 v18.4,12.6 C30.1
CMD3+  (via drill 0.3)
  Top 0.15: U$3.CMD+(95) 85.25,53.35 86.2,54.3 v88.1,54.3
  Top 0.3: R73.2 83.1,67.8 v82.9,68
  Bottom 0.15: R61.1 89.9,39.4 88.8,40.5 88.8,53.6 v88.1,54.3 86.6,55.8 86.6,61.9 83,65.5 83,66.95 R66.1 82.9,66.95
  Bottom 0.3: C33.1 83,68.1 v82.9,68 82.9,67.05 R66.1
CMD3-  (via drill 0.3)
  Top 0.15: U$3.CMD-(94) 85.45,53.05 86.1,53.7 v87.5,53.7
  Top 0.3: R74.2 v81.6,68
  Bottom 0.15: R62.1 88.4,52.8 v87.5,53.7 86.25,54.95 86.25,61.65 81.65,66.25 R66.2
  Bottom 0.3: C34.1 v81.6,68 81.6,67.05 R66.2
CMD4+  (via drill 0.3)
  Top 0.15: U$4.CMD+(95) 85.25,33.35 86.2,34.3 v88.1,34.3 | R59.1 51.2,10 52.4,11.2 60.1,11.2 64.2,7.1 76.9,7.1 80.3,10.5 82.5,10.5 v84.5,12.5
  Top 0.3: R71.2 v84.5,12.5
  Bottom 0.15: R61.2 89.9,36.7 89.6,36.4 89,36.4 88.1,35.5 v88.1,34.3 89.3,33.1 89.3,18.9 85.5,15.1 84.8,15.1 84.35,14.65 R65.1
  Bottom 0.3: R65.1 84.5,13.65 v84.5,12.5 84.5,11.45 C31.1
CMD4-  (via drill 0.3)
  Top 0.15: U$4.CMD-(94) 85.45,33.05 86.1,33.7 v87.5,33.7 | R60.1 60.3,11.6 64.4,7.5 76.7,7.5 80.1,10.9 81.5,10.9 v83.1,12.5
  Top 0.3: v83.1,12.5 R72.2
  Bottom 0.15: R62.2 88.4,36.7 87.5,35.8 v87.5,33.7 88.9,32.3 88.9,19.1 85.3,15.5 83.8,15.5 83.1,14.8 83.1,13.85 R65.2
  Bottom 0.3: R65.2 83.1,13.75 v83.1,12.5 C32.1
DOB1+  (via drill 0.3)
  Top 0.15: U$1.DOB+(103) 14.85,46.25 14.2,45.6 v11.2,45.6
  Bottom 0.15: v11.2,45.6 10.2,46.6 10.2,62 14.5,66.3 14.5,67.6 13.6,68.5 C55.2
DOB1-  (via drill 0.3)
  Top 0.15: U$1.DOB-(104) 15.05,45.95 14.1,45 v10.6,45
  Bottom 0.15: v10.6,45 9.8,45.8 9.8,62.1 14.1,66.4 14.1,67.4 13.2,68.3 12.5,68.3 12.2,68.6 C56.2
DOB2+  (via drill 0.3)
  Top 0.15: U$2.DOB+(103) 14.85,26.25 14.2,25.6 v11.2,25.6
  Bottom 0.15: v11.2,25.6 11.7,25.1 11.7,18.9 15.8,14.8 15.8,12.8 15.2,12.2 C57.2
DOB2-  (via drill 0.3)
  Top 0.15: U$2.DOB-(104) 15.05,25.95 14.1,25 v10.6,25
  Bottom 0.15: v10.6,25 11.3,24.3 11.3,18.7 15.4,14.6 15.4,13.1 14.6,12.3 14,12.3 13.7,12 C58.2
DOB3+  (via drill 0.3)
  Top 0.15: U$3.DOB+(103) 85.15,54.15 85.9,54.9 v88.7,54.9
  Bottom 0.15: v88.7,54.9 87.45,56.15 87.45,62.3 83.8,65.95 83.8,67.9 84.4,68.5 C59.2
DOB3-  (via drill 0.3)
  Top 0.15: U$3.DOB-(104) 84.95,54.45 86,55.5 v89.3,55.5
  Bottom 0.15: v89.3,55.5 87.9,56.9 87.9,62.4 84.2,66.1 84.2,67.7 84.8,68.3 85.5,68.3 85.8,68.6 C60.2
DOB4+  (via drill 0.3)
  Top 0.15: U$4.DOB+(103) 85.15,34.15 85.9,34.9 v88.7,34.9
  Bottom 0.15: v88.7,34.9 90,33.6 90,18.4 86.2,14.6 C61.2
DOB4-  (via drill 0.3)
  Top 0.15: U$4.DOB-(104) 84.95,34.45 86,35.5 v89.3,35.5
  Bottom 0.15: v89.3,35.5 90.4,34.4 90.4,18.3 87.7,15.6 C62.2
GND  (via drill 0.3, 0.3 pad 0.7, 0.9, 1 pad 1.78)
  Top 0.3: v18.6,64.8 R49.1 | R51.1 20.4,14.95 20.4,15.5 20.9,16 v21.7,16 | R29.1 R91.1 | R53.1 81.4,15.4 81,15.8 v80.5,15.8 | 20.55,61.05 C35.2 20.55,60.95 21,60.5 21,59.8 v21.2,59.6 | C36.2 20.55,41.35 | 20.55,41.05 C36.2 | R67.1 15.5,64.05 C51.1 | v78.8,57.6 79,57.6 79,58.6 79.45,59.05 C43.2 | v21.2,42.8 21,42.6 21,41.7 20.55,41.25 | v21.2,39.6 21,39.8 21,40.7 20.55,41.15 C36.2 | v78.8,37.6 79,37.8 79,38.7 79.45,39.15 | v78.8,40.8 79,40.6 79,39.7 79.45,39.25 C44.2 | C54.1 83.05,65.6 R73.1 | v78.8,48.8 U$3.GND | U$4.GND v78.8,28.8 | U$2.GND v21.2,30.8
  Top 0.5: R10.1 v15.9,56.6 | R19.1 v15.9,36.6 | R37.1 v84.1,23.7 | C53.1 v78.6,12.5 | R28.1 v84,43.8 | R20.1 v15.9,37.9 | R92.1 v15.9,39.1 | R90.1 v15.9,59.2 | R11.1 v15.9,57.9 | R29.1 v84,42.5 | R38.1 v84.1,22.4 | R93.1 v84.1,21.1 | C52.1 v23.2,12.6 | R69.1 15.15,14.85 v14.6,14.3 | C2.2 v57.6,69.3 | C1.2 v35.9,69.3 | C40.2 v21.9,18.4 | C41.2 v17.3,40.5 | C38.2 v17.3,42 | v15.8,62.6 15.55,62.85 C51.1 | C39.2 v14.7,57.6 | C50.2 v81.6,18.4 | C45.2 v82.9,58.4 | C46.2 v82.9,40 | C49.2 v82.9,38.4 | R55.1 v80,64.8 | C54.1 83.05,63.55 v82.3,62.8 | C37.2 v17.3,60.5 | v21.2,50.8 U$1.GND | R85.1 v54.7,90.6 | C47.2 v85.3,42.7 | C48.2 78.05,17.1 v77,17.1 | R71.1 v84.5,17.5 | C42.2 v18.4,20.4 | C65.2 v14.7,37.7 | C66.2 v85.7,21.9
  Top 1: C64.- v61.3,77.9 | C63.- 61.8,67 v61.8,64.9
  other vias: 52.55,97.55 52.55,92.45 47.45,97.55 47.45,92.45 21.2,44.4 21.2,43.6 21.2,45.2 21.2,46 21.2,46.8 21.2,47.6 21.2,48.4 21.2,51.6 21.2,50 21.2,49.2 21.2,58.8 21.2,58 21.2,57.2 21.2,56.4 21.2,55.6 21.2,54.8 21.2,54 21.2,53.2 21.2,52.4 21.2,22.8 21.2,24.4 21.2,23.6 21.2,25.2 21.2,26 21.2,26.8 21.2,27.6 21.2,28.4 21.2,31.6 21.2,30 21.2,29.2 21.2,38.8 21.2,38 21.2,37.2 21.2,36.4 21.2,35.6 21.2,34.8 21.2,34 21.2,33.2 21.2,32.4 78.8,42.4 78.8,41.6 78.8,43.2 78.8,44 78.8,44.8 78.8,45.6 78.8,46.4 78.8,49.6 78.8,48 78.8,47.2 78.8,56.8 78.8,56 78.8,55.2 78.8,54.4 78.8,53.6 78.8,52.8 78.8,52 78.8,51.2 78.8,50.4 78.8,20.8 78.8,22.4 78.8,21.6 78.8,23.2 78.8,24 78.8,24.8 78.8,25.6 78.8,26.4 78.8,29.6 78.8,28 78.8,27.2 78.8,36.8 78.8,36 78.8,35.2 78.8,34.4 78.8,33.6 78.8,32.8 78.8,32 78.8,31.2 78.8,30.4
  pour Bottom: 0.1,99.9 0.1,0.1 99.9,0.1 99.9,99.9 48.5,99.9 48.5,89.2 50,87.7 50,78 48.5,76.5 41,76.5 39.5,78 39.5,87.7 41,89.2 48.4,89.2 48.4,99.9
HITOR  (via drill 0.3, 1 pad 1.78)
  Top 0.15: R81.2 84.9,55.3 87.2,57.6 v88.5,57.6 | R79.2 15.2,45.1 10.45,40.35 v10.45,39.25 | 16.1,25.1 R80.2 15.6,25.1 14.05,23.55 v9.85,23.55 | R82.2 84.8,35.3 85.8,36.3 v90.9,36.3 | v64.8,90.6 74.1,90.6 75.6,89.1 75.6,82.8 87,71.4 87,62.9 v88.5,61.4 | v62.2,90.6 R85.2 | v9.85,21.1 9.85,17.15 17.5,9.5 20.7,9.5 24,6.2 77.1,6.2 80.7,9.8 82.9,9.8 90.2,17.1 90.2,33 v92.2,35
  Top 0.3: R85.2 57.65,91.35 57.1,91.9 55.4,91.9 53.8,93.5 v53.8,95
  Bottom 0.15: v64.8,90.6 v62.2,90.6 | v10.45,39.25 9.4,38.2 9.4,24 v9.85,23.55 v9.85,21.1 | v88.5,61.4 v88.5,57.6 90.1,56 90.1,54.4 89.3,53.6 89.3,40.9 90.9,39.3 v90.9,36.3 v92.2,35
  Bottom 0.3: v50,95 v53.8,95
N$1
  Top 0.5: BACKPLANE.TP 50.02,64.72 R2.2 C2.1
N$2
  Top 0.5: C1.1 43.68,69.3 R1.2 47.16,69.28 R2.1
N$3  (via drill 0.3)
  Top 0.15: v25.8,89.5 23.4,91.9 13.13,91.9 9.6,88.37 9.6,85.9 9,85.3 7.03,85.3 JP13.2 | U$17.P$1 35.8,63.3 36,63.5 36,64 35.8,64.2 35.2,64.2 34.8,64.6 34.8,73.4 30,78.2 v29,78.2
  Bottom 0.15: v25.8,89.5 25.8,86.4 28.6,83.6 28.6,78.6 v29,78.2
N$4  (via drill 0.3)
  Top 0.15: U$1.RESET1(45) 19.35,54.95 v19,55.3 18.25,55.3 R3.1
  Bottom 0.15: C3.1 v19,55.3
N$5  (via drill 0.3)
  Top 0.15: U$1.RESET2(56) v19,53.2 R4.1
  Bottom 0.15: v19,53.2 18.25,53.2 C4.1
N$6  (via drill 0.3)
  Top 0.15: U$1.RESET3(88) 19.65,48.65 19.6,48.7 19.6,49.1 v19,49.7 18.7,50 18.05,50 R5.1
  Bottom 0.15: C5.1 18.25,50 18.7,50 v19,49.7
N$7  (via drill 0.3)
  Top 0.15: U$1.RESET4(89) 19.35,48.35 v19,48.7 18.25,48.7 R6.1
  Bottom 0.15: C6.1 18.15,48.7 v19,48.7
N$8
  Top 0.15: U$1.GA0(67) 19.6,51.7 19.2,52.1 15.9,52.1 15.3,52.7 14.95,52.7 R7.1
N$9
  Top 0.15: U$1.GA1(68) 19.45,51.35 19,51.8 14.95,51.8 R8.1
N$10
  Top 0.15: U$1.GA2(69) 19.3,51 18.8,51.5 16.7,51.5 15.5,50.3 R9.1
N$11
  Top 0.15: U$1.IREF(33,34) 18.2,56.55 R10.2
N$12
  Top 0.15: U$1.VTHR(24,16) 19.2,58.3 18.8,57.9 R11.2
N$13
  Top 0.15: U$1.HITOR(105) 19.35,45.55 18.9,45.1 R79.1
N$14
  Top 0.15: U$2.GA0(67) 19.5,31.7 19.2,32 15.8,32 15.4,32.4 14.85,32.4 R16.1 14.95,32.3
N$15
  Top 0.15: U$2.GA1(68) 19.35,31.35 19,31.7 15.9,31.7 15.4,31.2 R17.1 14.85,31.3
N$16
  Top 0.15: U$2.GA2(69) 19.2,31 18.8,31.4 16.2,31.4 15.5,30.7 15.5,30 15.3,29.8 R18.1 14.95,30
N$17  (via drill 0.3)
  Top 0.15: U$2.RESET1(45) 19.35,34.95 v19,35.3 C7.1 R12.1
  Bottom 0.15: C7.1 v19,35.3
N$18  (via drill 0.3)
  Top 0.15: U$2.RESET2(56) v19,33.2 R13.1
  Bottom 0.15: C8.1 R13.1 v19,33.2
N$19  (via drill 0.3)
  Top 0.15: U$2.RESET3(88) 19.65,28.65 19.6,28.7 19.6,29.1 v19,29.7 18.7,30 18.45,30 R14.1
  Bottom 0.15: C9.1 18.15,30 18.7,30 v19,29.7
N$20  (via drill 0.3)
  Top 0.15: U$2.RESET4(89) 19.35,28.35 v19,28.7 18.35,28.7 R15.1
  Bottom 0.15: C10.1 18.25,28.7 v19,28.7
N$21
  Top 0.15: U$2.HITOR(105) 19.55,25.55 19.1,25.1 R80.1
N$22
  Top 0.15: U$3.HITOR(105) 80.65,54.85 81.1,55.3 R81.1
N$23
  Top 0.15: U$4.HITOR(105) 80.75,34.85 81.1,35.2 81.75,35.2 R82.1
N$24
  Top 0.15: U$1.TDAC(11) 18.15,59.15 R90.2
N$25
  Top 0.15: U$2.IREF(33,34) 18.2,36.55 R19.2
N$26
  Top 0.15: U$2.VTHR(24,16) 19.4,38.3 19.1,38 18.25,38 R20.2
N$27
  Top 0.15: U$3.TDAC(11) 81.8,41.25 R91.2
N$28
  Top 0.15: U$2.TDAC(11) 18.2,39.15 R92.2
N$29
  Top 0.15: U$4.TDAC(11) 81.7,21.25 R93.2
N$30  (via drill 0.3)
  Top 0.15: v28.2,77.3 30.3,77.3 34.4,73.2 34.4,63.9 34.5,63.8 U$17.P$2 | v24.6,89.5 22.6,91.5 13.3,91.5 10,88.2 10,83.8 9,82.8 7.07,82.8 JP13.1
  Bottom 0.15: v28.2,77.3 28.2,83.5 25.4,86.3 25.4,88.7 v24.6,89.5
N$31
  Top 0.15: U$18.P$2 65.4,63.8 65.4,77 61.8,80.6 61.8,88.7 64.6,91.5 86.8,91.5 89.5,88.8 89.5,84.1 90.77,82.83 JP14.1
N$32
  Top 0.15: U$18.P$1 64.2,63.3 64,63.5 64,64 64.3,64.3 64.7,64.3 65,64.6 65,76.9 61.4,80.5 61.4,88.8 64.5,91.9 87.1,91.9 90,89 90,86 90.63,85.37 JP14.2
N$34
  Top 0.5: X1.1 R1.1
N$46  (via drill 0.3)
  Top 0.15: U$21.P$2 25.1,17.1 24.7,16.7 24.7,11.6 v24.3,11.2 | v22.7,5.1 11.9,5.1 9.7,7.3 9.7,11.2 4.2,16.7 4.2,65.7 7.9,69.4 7.9,74.6 9.3,76 9.3,77.8 7.93,79.17 JP9.1
  Bottom 0.15: v24.3,11.2 24.3,6.7 v22.7,5.1
N$47  (via drill 0.3)
  Top 0.15: U$21.P$1 25.3,16.6 25.1,16.4 v25.1,10.4 | v23.3,4.4 22.3,4.4 22,4.7 11.7,4.7 9.3,7.1 9.3,11.1 3.8,16.6 3.8,65.9 7.5,69.6 7.5,76.13 JP9.2
  Bottom 0.15: v25.1,10.4 25.1,6.2 v23.3,4.4
N$48  (via drill 0.3)
  Top 0.15: U$22.P$2 75.2,17.1 76.1,16.2 76.1,10.5 v76.5,10.1 | v78.9,6.7 86.9,6.7 96.8,16.6 96.8,64.2 92,69 92,74.7 90.9,75.8 90.9,78.1 92.07,79.27 JP10.1
  Bottom 0.15: v76.5,10.1 76.5,8.4 78.2,6.7 v78.9,6.7
N$49  (via drill 0.3)
  Top 0.15: U$22.P$1 75,16.6 75.7,15.9 v75.7,9.5 | v78.2,6 86.8,6 97.2,16.4 97.2,64.4 92.5,69.1 92.5,76.33 JP10.2
  Bottom 0.15: v75.7,9.5 75.7,8.5 v78.2,6
N$50
  Top 0.15: U$3.GA2(69) 80.8,49.4 81.2,49 83.3,49 84.7,50.4 84.95,50.4 R27.1
N$56
  Top 0.15: U$3.IREF(33,34) 81.8,43.85 R28.2
N$57
  Top 0.15: U$3.GA1(68) 80.65,49.05 81.1,48.6 83.5,48.6 84.1,49.2 85.15,49.2 R26.1
N$58
  Top 0.15: U$3.GA0(67) 80.5,48.7 81,48.2 84.2,48.2 84.6,47.8 85.15,47.8 R25.1 85.05,48.1
N$59  (via drill 0.3)
  Top 0.15: U$3.RESET1(45) 80.65,45.45 v81,45.1 C11.1 R21.1
  Bottom 0.15: C11.1 v81,45.1
N$60  (via drill 0.3)
  Top 0.15: U$3.RESET2(56) v81,47.2 R22.1 C12.1
  Bottom 0.15: C12.1 R22.1 v81,47.2
N$61  (via drill 0.3)
  Top 0.15: U$3.RESET3(88) 80.35,51.75 80.4,51.7 80.4,51.3 v81,50.7 81.4,50.3 R23.1
  Bottom 0.15: C13.1 81.3,50.4 v81,50.7
N$62  (via drill 0.3)
  Top 0.15: U$3.RESET4(89) 80.75,52.05 v81,51.8 81.65,51.8 R24.1
  Bottom 0.15: C14.1 81.75,51.8 v81,51.8
N$64
  Top 0.15: U$3.VTHR(24,16) 80.8,42.1 81.1,42.4 81.75,42.4 R29.2
N$73
  Top 0.15: R34.1 85.15,27.6 84.6,27.6 83.9,28.3 80.8,28.3 80.4,28.7 U$4.GA0(67)
N$74
  Top 0.15: R35.1 85.05,28.6 81,28.6 80.55,29.05 U$4.GA1(68)
N$75
  Top 0.15: R36.1 84.95,29.8 84.7,29.8 83.8,28.9 81.2,28.9 80.7,29.4 U$4.GA2(69)
N$76  (via drill 0.3)
  Top 0.15: U$4.RESET1(45) 80.65,25.45 v81,25.1 C15.1 R30.1
  Bottom 0.15: C15.1 v81,25.1
N$77  (via drill 0.3)
  Top 0.15: U$4.RESET2(56) v81,27.2 R31.1
  Bottom 0.15: C16.1 R31.1 v81,27.2
N$78  (via drill 0.3)
  Top 0.15: U$4.RESET3(88) 80.35,31.75 80.4,31.7 80.4,31.3 v81,30.7 81.3,30.4 81.85,30.4 R32.1
  Bottom 0.15: C17.1 81.65,30.4 81.3,30.4 v81,30.7
N$79  (via drill 0.3)
  Top 0.15: U$4.RESET4(89) 80.65,32.05 v81,31.7 81.65,31.7 R33.1
  Bottom 0.15: C18.1 81.1,31.6 v81,31.7
N$80
  Top 0.15: U$4.IREF(33,34) 81.7,23.85 R37.2
N$81
  Top 0.15: U$4.VTHR(24,16) 80.8,22.1 81,22.3 81.75,22.3 R38.2
NTC1+
  Top 0.15: J1.2-3 31.33,89.9 36.6,89.9 38,88.5 38,84.4 36.7,83.1 35.9,83.1 34.47,81.67 JP5.1
NTC1-
  Top 0.15: J1.2-6 35.18,87.4 36.8,87.4 37.6,86.6 37.6,84.7 36.5,83.6 34.1,83.6 31.9,81.4 31.9,79.63 JP5.2
NTC2+
  Top 0.15: J1.1-3 17.36,89.9 23,89.9 24.5,88.4 24.5,84.33 23.97,83.8 JP6.1
NTC2-
  Top 0.15: J1.1-6 21.21,87.4 23.3,87.4 24,86.7 24,85.4 23.4,84.8 22.4,84.8 21.43,83.83 JP6.2
NTC3+
  Top 0.15: J2.1-3 67.46,90 72.3,90 74.1,88.2 74.1,81.77 JP7.1
NTC3-
  Top 0.15: J2.1-6 71.21,87.4 73,87.4 73.6,86.8 73.6,85.2 73.1,84.7 72,84.7 71.6,84.3 71.6,81.73 JP7.2
NTC4+
  Top 0.15: J2.2-3 81.53,90.1 86.5,90.1 88.3,88.3 88.3,81.77 JP8.1
NTC4-
  Top 0.15: J2.2-6 85.18,87.4 87.1,87.4 87.8,86.7 87.8,85.4 87.2,84.8 86.3,84.8 85.8,84.3 85.8,81.73 JP8.2
VDDA  (via drill 0.3, 0.3 pad 0.7)
  Top 0.3: R3.2 v15.9,55.4 15.85,55.45 C39.1 | R12.2 v13.4,35.4 14.65,35.4 C65.1 14.75,35.4 | C35.1 U$1.VDDA C36.1 U$2.VDDA v21.85,21.5 21.85,20.7 C40.1 | 21.85,63.35 v21.8,63.2 | v19.7,63.2 17.9,63.2 13.5,58.8 13.5,55.8 13.85,55.45 C39.1 | 14.65,55.4 C39.1 | C43.1 U$3.VDDA C44.1 U$4.VDDA v78.15,19.45 78.1,19.55 | v80.4,20.6 81.2,19.8 85.3,19.8 87.1,21.6 v87.1,24.2 85.65,24.2 | R21.2 85.35,45 | R13.2 16,33.2 15.6,33.6 v13.4,33.6 12.9,33.6 12.15,32.85 12.15,28 9.05,24.9 9.05,22.9 10.45,21.5 v19.85,21.5 | R22.2 83.8,47.2 84.3,46.7 v86.6,46.7 87.2,46.7 87.6,47.1 87.6,52.3 90.2,54.9 90.2,59 88.9,60.3 v81.85,60.3 | 85.2,45.05 C47.1 85.35,45 | R31.2 84,27.2 85.3,25.9 v87.1,25.9 | R30.2 84.1,25 84.9,24.2 85.65,24.2 | 85.65,24.2 C66.1 | 85.35,45 v86.6,45
  Top 0.5: R4.2 v15.9,53.2 | C35.1 21.85,63.2 v21.8,63.2 | C43.1 v78.15,60.3 | 78.1,19.55 C48.1
  Top 1: v78.15,60.3 78.15,62.25 74.6,65.8 74.6,69.6 v71.9,72.3 v71.1,72.3 v70.3,72.3 v69.5,72.3 v68.7,72.3 | v31,72.3 v30.2,72.3 v29.4,72.3 v28.6,72.3 v27.8,72.3 24.9,69.4 24.9,66.4 21.85,63.35 | v61.6,72.3 v62.4,72.3 v63.2,72.3 | v61.6,72.3 v60.8,72.3 v60,72.3 56.9,72.3 52.1,77.1 X1.3 | C63.+ 61.6,70 v61.6,72.3
  Bottom 0.3: v15.9,55.4 v15.9,53.2 | v19.7,63.2 v21.8,63.2 | v13.4,33.6 v13.4,35.4 | v86.6,45 v86.6,46.7 | v87.1,24.2 v87.1,25.9 | v19.85,21.5 v21.85,21.5 | v78.15,60.3 v81.85,60.3
  Bottom 0.5: v78.15,19.45 79.25,19.45 v80.4,20.6
  Bottom 1: v27.8,72.3 v63.2,72.3 v68.7,72.3 v71.9,72.3
VDDD  (via drill 0.3 pad 0.7)
  Top 0.15: R23.2 83.15,49.65 82.9,49.4 81.3,49.4 80.9,49.8 79.45,49.8 | R32.2 83.15,29.45 83,29.3 81.3,29.3 80.7,29.9 79.45,29.9 U$4.VDDD | R5.2 16.85,50.95 17.1,51.2 18.6,51.2 19.3,50.5 20.55,50.5 | R14.2 16.85,30.95 17,31.1 18.6,31.1 19.2,30.5 20.55,30.5 20.55,30.2
  Top 0.3: U$3.VDDD 79.45,40.1 80.35,40.1 C46.1 C49.1 80.55,38.3 79.45,38.3 79.45,29.9 | R23.2 R24.2 86.3,51.6 86.5,51.4 86.5,50.75 R27.2 R26.2 R25.2 | U$3.VDDD 79.45,49.8 | R32.2 R33.2 86.2,31.5 86.55,31.15 R36.2 R35.2 R34.2 | R54.1 C53.2 78.6,15.7 79.5,16.6 | R72.1 83.1,15.8 82.3,16.6 79.5,16.6 | R7.2 R8.2 R9.2 13.4,50.25 13.4,49.2 13.8,48.8 16.75,48.8 R6.2 R5.2 | R50.1 20.05,65.6 20.05,64.85 | R16.2 R17.2 R18.2 13.45,29.05 13.7,28.8 16.75,28.8 R15.2 R14.2 | 21.65,14.9 R52.1 C52.2 23.2,16.4 22.3,17.3 20.5,17.3 | 20.5,17.3 19.5,17.3 18.4,16.2 R70.1 | 78.4,65.55 R56.1 78.7,65.45 78.7,64.9 79.6,64 | C37.1 19.45,59.7 19.65,59.5 20.55,59.5 U$1.VDDD 20.55,50.5 20.55,42.2 19.65,42.2 C38.1 C41.1 19.5,40.45 19.5,39.8 19.75,39.55 20.55,39.55 U$2.VDDD 20.55,30.2 C42.1 20.55,17.35 20.5,17.3 | C51.2 16.8,64.05 R68.1 | C51.2 19.2,64 20.05,64.85 | 16.8,63.95 C51.2 | U$4.VDDD C50.1 79.45,16.65 79.5,16.6 | U$3.VDDD 79.45,58.3 80.65,58.3 C45.1 80.8,58.4 80.8,59.2 | 20.05,64.85 20.65,64.25 20.75,64.25 | R74.1 81.75,65.5 C54.2 81.65,64 79.6,64 | 79.6,64 78.95,63.35
  Top 0.5: C37.1 19.45,61.65 20.75,62.95 20.75,64.25 | 80.8,59.8 80.75,59.75 C45.1
  Top 1: 20.75,64.25 23.5,67 23.5,69.9 27.2,73.6 v29.4,73.6 v30.2,73.6 v31,73.6 v31.8,73.6 | v67.9,73.6 v68.7,73.6 v69.5,73.6 v70.3,73.6 v71.1,73.6 72.5,73.6 75.9,70.2 75.9,66.4 78.95,63.35 80.8,61.5 80.8,59.8 | X1.4 C64.+
  Bottom 1: 56.3,73.6 v31.8,73.6 v28.6,73.6 | 56.3,73.6 X1.4 | v71.1,73.6 v67.9,73.6 56.3,73.6

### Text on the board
Top: Hit | OR | C | T | T | C | T1 | T3 | T4 | T2 | V | V | HV | Liverpool University I.T. May 2013 | Quad Pixel Rigid Board V2.1
tValues: + | +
